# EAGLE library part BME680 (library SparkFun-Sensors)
Bosch BME680 &ndash; Combined Humidity and Pressure Sensor The BME680 is as combined digital humidity, pressure and temperature sensor based on proven sensing principles. The sensor module is housed in an extremely compact metal-lid LGA package with a footprint of only 3.0×3.0mm with a height of 0.93mm. Its small dimensions and its low power consumption allow the implementation in battery driven devices such as handsets, GPS modules or watches.
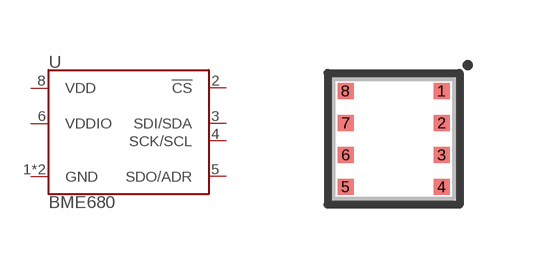
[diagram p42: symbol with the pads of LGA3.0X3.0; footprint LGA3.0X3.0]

Designator prefix U

## BME680-LGA (PROD_ID: IC-14656; VALUE: BME680)  [LGA3.0X3.0]
1  GND
2  !CS
3  SDI/SDA
4  SCK/SCL
5  SDO/ADR
6  VDDIO
7  GND
8  VDD

## Footprint LGA3.0X3.0 (pad centres in mm)
smd 0.4 x 0.4: 1 1.2,1.2; 2 1.2,0.4; 3 1.2,-0.4; 4 1.2,-1.2; 5 -1.2,-1.2; 6 -1.2,-0.4; 7 -1.2,0.4; 8 -1.2,1.2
